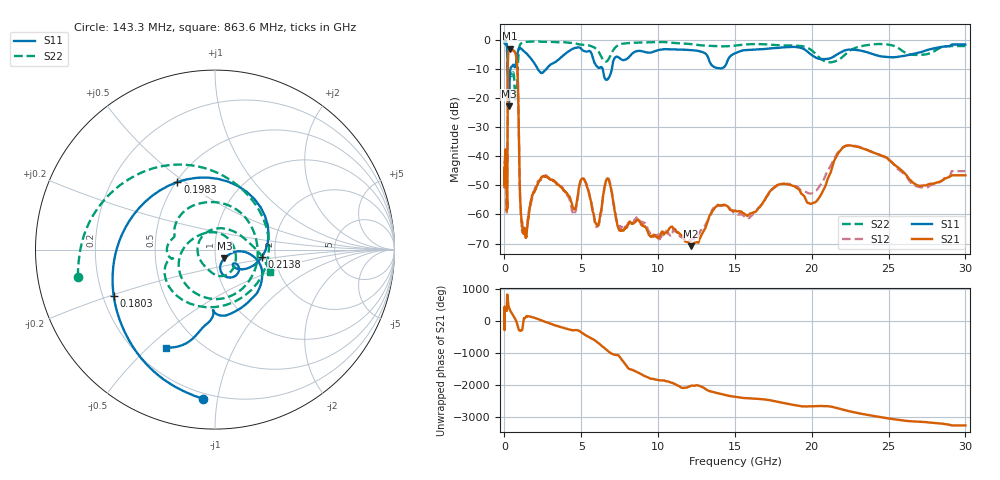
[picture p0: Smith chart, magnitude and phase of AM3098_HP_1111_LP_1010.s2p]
! Date/Time: Thu, Feb 28, 2019 8:48 AM
! Network Analyzer: Agilent Technologies E8364B Rev: A.07.50.67
! Sweep from 0.010 to 30.000 GHz, 1601 Points, Sweep Type: LOG
! Power Supply: 5.022 V, 0.002 A
# Hz S DB R 50
!freq MagS11 AngS11 MagS21 AngS21 MagS12 AngS12 MagS22 AngS22
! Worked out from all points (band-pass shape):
!   1601 points, 10 MHz to 30 GHz, reference 50 ohm
!   highest |S21| = -3.09 dB at 340.5 MHz (marker M1); lowest = -70.9 dB at 12.13 GHz (marker M2)
!   |S21| within 3 dB of the highest: 228.4 MHz to 773 MHz (544.6 MHz wide, 109 % of centre)
!   lowest |S11| = -22.8 dB at 293 MHz (marker M3), VSWR 1.16, Z = 55.3 - j5.48 ohm
!   |S11| at or under -10 dB: 210.1 MHz to 390.2 MHz (180.1 MHz wide, 60 % of centre); 2.156 GHz to 2.736 GHz (579.7 MHz wide, 23.7 % of centre); 6.386 GHz to 6.99 GHz (603.4 MHz wide, 9.02 % of centre)
!   |S22| runs from -20.6 to -0.6 dB; largest |S21 - S12| = 0.011
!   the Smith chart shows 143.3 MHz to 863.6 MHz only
!   S11 on the Smith chart (normalised r, x): 143.3 MHz: 0.17, -0.91; 180.3 MHz: 0.24, -0.20; 198.3 MHz: 0.51, +0.47; 213.8 MHz: 1.71, -0.14; 863.6 MHz: 0.33, -0.57
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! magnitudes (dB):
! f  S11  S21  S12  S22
! 10 MHz  -0.4  -44.9  -44.1  -0.6
! 38.04 MHz  -0.2  -41.2  -40.8  -0.7
! 99.92 MHz  -0.9  -39.4  -39.0  -1.5
! 143.3 MHz  -1.6  -55.0  -54.4  -2.2
! 144.7 MHz  -1.6  -55.7  -54.8  -2.2
! 180.3 MHz  -4.2  -58.0  -55.8  -5.4
! 198.3 MHz  -7.3  -36.4  -36.5  -10.4
! 213.8 MHz  -11.5  -12.8  -12.8  -9.6
! 293 MHz  -22.8  -3.3  -3.2  -12.3
! 340.5 MHz  -12.9  -3.1  -3.1  -11.8
! 550.5 MHz  -8.7  -3.6  -3.6  -11.3
! 863.6 MHz  -4.3  -12.6  -12.6  -9.7
! 1.132 GHz  -3.2  -62.7  -64.2  -1.1
! 2.084 GHz  -9.3  -50.5  -49.6  -0.6
! 5.128 GHz  -3.7  -47.7  -47.5  -1.7
! 6.019 GHz  -9.1  -63.8  -64.3  -3.4
! 6.719 GHz  -13.6  -47.7  -47.6  -7.1
! 7.926 GHz  -6.7  -64.3  -64.1  -1.2
! 12.13 GHz  -3.5  -70.9  -68.9  -1.5
! 20.1 GHz  -5.6  -56.0  -52.6  -4.1
! 22.56 GHz  -3.4  -36.3  -36.1  -3.5
! 30 GHz  -1.6  -46.6  -45.1  -2.2
